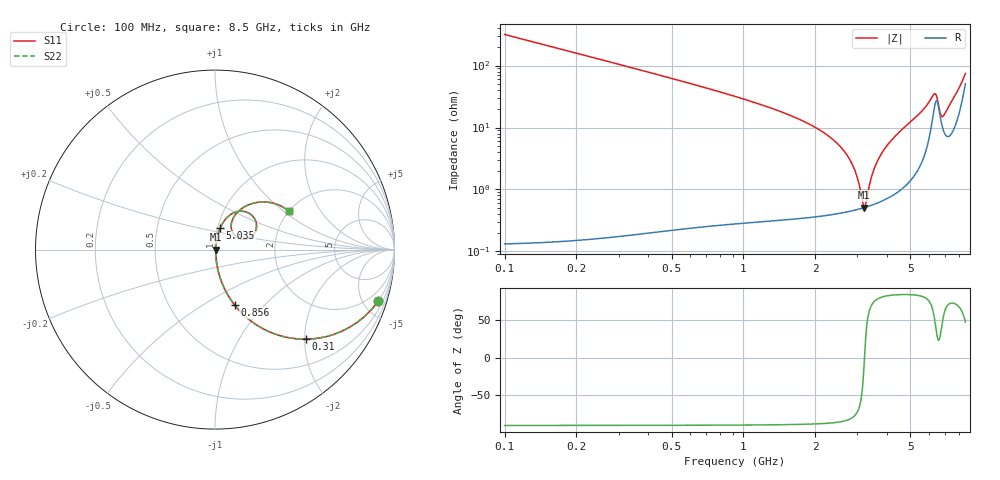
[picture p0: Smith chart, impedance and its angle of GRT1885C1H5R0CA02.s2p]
!Murata Part Number: GRT1885C1H5R0CA02
!These Parameters are Measured in Series Mode Connection
!Data Generated on Jun 19, 2026
!  o--ll--o
!Port1  Port2
!  o------o
!Operation Temp=25[degC], DC Bias Voltage=0[V]
!Freq. Start=100[MHz] Stop=9[GHz] 401[Steps]
# Hz S RI R 50
!Freq.(Hz) S11(Real) S11(Imag) S21(Real) S21(Imag) S12(Real) S12(Imag) S22(Real) S22(Imag)
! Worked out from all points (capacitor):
!   401 points, 100 MHz to 8.5 GHz, reference 50 ohm
!   read as one part in series: C = 5 pF near 142 MHz
!   lowest |Z| = 511 mohm at 3.208 GHz (marker M1)
!   series resonance near 3.213 GHz, so ESL is about 490 pH
!   S11 on the Smith chart (normalised r, x): 100 MHz: 1.00, -6.36; 310 MHz: 1.00, -2.03; 856 MHz: 1.01, -0.69; 5.035 GHz: 1.03, +0.25; 8.5 GHz: 2.01, +1.09
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1e8  0.9099 -0.2861  0.0901 0.2861  0.0901 0.2861  0.9099 -0.2861
2.05e8  0.7049 -0.4556  0.2951 0.4556  0.2951 0.4556  0.7049 -0.4556
3.1e8  0.5085 -0.4991  0.4915 0.4991  0.4915 0.4991  0.5085 -0.4991
5.41e8  0.2475 -0.4296  0.7525 0.4296  0.7525 0.4296  0.2475 -0.4296
8.56e8  0.1092 -0.308  0.8908 0.308  0.8908 0.308  0.1092 -0.308
1.507e9  0.0302 -0.1617  0.9698 0.1617  0.9698 0.1617  0.0302 -0.1617
2.431e9  0.00738 -0.058  0.9926 0.058  0.9926 0.058  0.00738 -0.058
2.914e9  0.00502 -0.0206  0.995 0.0206  0.995 0.0206  0.00502 -0.0206
3.208e9  0.00507 -0.000326  0.9949 0.000326  0.9949 0.000326  0.00507 -0.000326
3.25e9  0.00515 0.00247  0.9948 -0.00247  0.9948 -0.00247  0.00515 0.00247
3.439e9  0.00575 0.0148  0.9943 -0.0148  0.9943 -0.0148  0.00575 0.0148
3.607e9  0.00657 0.0256  0.9934 -0.0256  0.9934 -0.0256  0.00657 0.0256
3.901e9  0.00871 0.0441  0.9913 -0.0441  0.9913 -0.0441  0.00871 0.0441
4.3e9  0.0132 0.0692  0.9868 -0.0692  0.9868 -0.0692  0.0132 0.0692
5.035e9  0.0288 0.1197  0.9712 -0.1197  0.9712 -0.1197  0.0288 0.1197
5.707e9  0.0675 0.1793  0.9325 -0.1793  0.9325 -0.1793  0.0675 0.1793
6.295e9  0.213 0.1831  0.787 -0.1831  0.787 -0.1831  0.213 0.1831
6.526e9  0.1962 0.0685  0.8038 -0.0685  0.8038 -0.0685  0.1962 0.0685
6.736e9  0.1151 0.0742  0.8849 -0.0742  0.8849 -0.0742  0.1151 0.0742
7.114e9  0.0928 0.1528  0.9072 -0.1528  0.9072 -0.1528  0.0928 0.1528
7.996e9  0.2342 0.263  0.7658 -0.263  0.7658 -0.263  0.2342 0.263
8.5e9  0.4135 0.2127  0.5865 -0.2127  0.5865 -0.2127  0.4135 0.2127
